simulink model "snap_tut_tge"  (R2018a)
settings: Solver=VariableStepDiscrete  StartTime=0.0  StopTime=50000  RelTol=1e-3
undefined symbols (not defined in the file): bad_frame, Bit, Both, bram, c, cnt_rst, core_rst, d, data, data_in, eof, eof_in, Falling, hex2dec, ip, ip_in, led, led_rx, led_tx, led_up, link_up, Location, Lower, Minimum_Area, notused, out, overrun, reg, Rising, ROACH2, sfp, SNAP, tx_full, tx_over, Unsigned, Upper, valid, valid_in, Width, xc7k160t
libraries: xbsIndex_r4 x1201, casper_library_misc x9, xps_library x5
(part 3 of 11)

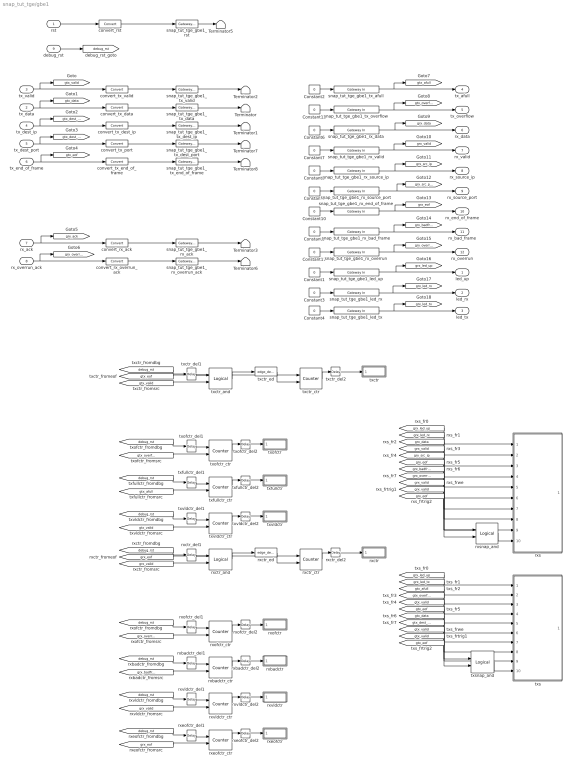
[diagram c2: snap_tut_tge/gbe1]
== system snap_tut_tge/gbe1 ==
  rst : Inport
  tx_data : Inport  Port=2
  tx_valid : Inport  Port=3
  tx_dest_ip : Inport  Port=4
  tx_dest_port : Inport  Port=5
  tx_end_of_frame : Inport  Port=6
  rx_ack : Inport  Port=7
  rx_overrun_ack : Inport  Port=8
  debug_rst : Inport  Port=9
  Constant{1..12} (12 alike) : Constant  Value=0
  Terminator{,1..3,5..8} (8 alike) : Terminator
  convert_rst : xbsIndex_r4/Convert  gui_display_data_type=Fixed-point  arith_type=Boolean  n_bits=64  bin_pt=0  float_type=Single  exp_bits=8  fraction_bits=24  quantization=Truncate  overflow=Wrap  en=off  latency=0  pipeline=off  dbl_ovrd=off  block_type=convert
  convert_rx_ack : xbsIndex_r4/Convert  gui_display_data_type=Fixed-point  arith_type=Boolean  n_bits=64  bin_pt=0  float_type=Single  exp_bits=8  fraction_bits=24  quantization=Truncate  overflow=Wrap  en=off  latency=0  pipeline=off  dbl_ovrd=off  block_type=convert
  convert_rx_overrun_ack : xbsIndex_r4/Convert  gui_display_data_type=Fixed-point  arith_type=Boolean  n_bits=64  bin_pt=0  float_type=Single  exp_bits=8  fraction_bits=24  quantization=Truncate  overflow=Wrap  en=off  latency=0  pipeline=off  dbl_ovrd=off  block_type=convert
  convert_tx_data : xbsIndex_r4/Convert  gui_display_data_type=Fixed-point  arith_type=Unsigned  n_bits=64  bin_pt=0  float_type=Single  exp_bits=8  fraction_bits=24  quantization=Truncate  overflow=Wrap  en=off  latency=0  pipeline=off  dbl_ovrd=off  block_type=convert
  convert_tx_dest_ip : xbsIndex_r4/Convert  gui_display_data_type=Fixed-point  arith_type=Unsigned  n_bits=32  bin_pt=0  float_type=Single  exp_bits=8  fraction_bits=24  quantization=Truncate  overflow=Wrap  en=off  latency=0  pipeline=off  dbl_ovrd=off  block_type=convert
  convert_tx_end_of_frame : xbsIndex_r4/Convert  gui_display_data_type=Fixed-point  arith_type=Boolean  n_bits=1  bin_pt=0  float_type=Single  exp_bits=8  fraction_bits=24  quantization=Truncate  overflow=Wrap  en=off  latency=0  pipeline=off  dbl_ovrd=off  block_type=convert
  convert_tx_port : xbsIndex_r4/Convert  gui_display_data_type=Fixed-point  arith_type=Unsigned  n_bits=16  bin_pt=0  float_type=Single  exp_bits=8  fraction_bits=24  quantization=Truncate  overflow=Wrap  en=off  latency=0  pipeline=off  dbl_ovrd=off  block_type=convert
  convert_tx_valid : xbsIndex_r4/Convert  gui_display_data_type=Fixed-point  arith_type=Boolean  n_bits=1  bin_pt=0  float_type=Single  exp_bits=8  fraction_bits=24  quantization=Truncate  overflow=Wrap  en=off  latency=0  pipeline=off  dbl_ovrd=off  block_type=convert
  rxbadctr : Subsystem  Tag=xps:sw_reg  AncestorBlock=xps_library/Memory/software_register  mask(swreg){io_dir=To Processor, io_delay=1, init_val=0, sample_period=1, names=reg, bitwidths=32, bin_pts=0, arith_types=0, sim_port=off, show_format=on}
      mask prompts: io_dir "I/O direction"; io_delay "I/O delay"; init_val "Initial Value"; sample_period "Sample period"; names "Bitfield names [msb...lsb]"; bitwidths "Bitfield widths"; bin_pts "Bitfield binary pts"; arith_types "Bitfield types, ufix=0, fix=1, bool=2"; sim_port "Provide sim input/output?"; show_format "Print format string?"
      mask help: A 32-bit software-accessible register. Can be divided into bitfields of varying widths and types using the fields in the block mask.
      mask init:
      | swreg_init(gcb)
  rxbadctr_ctr : xbsIndex_r4/Counter  cnt_type=Free Running  cnt_to=Inf  operation=Up  start_count=0  cnt_by_val=1  arith_type=Unsigned  n_bits=32  bin_pt=0  load_pin=off  rst=on  en=on  explicit_period=on  period=1  use_behavioral_HDL=on  implementation=Fabric  dbl_ovrd=off  block_type=counter
  rxbadctr_del1 : xbsIndex_r4/Delay  rst=off  infoeditControl=Selection of Reset will increase slice count due to use of real FFs and instead of SRLs  en=off  latency=2  reg_retiming=on  dbl_ovrd=off  block_type=delay
  rxbadctr_del2 : xbsIndex_r4/Delay  rst=off  infoeditControl=Selection of Reset will increase slice count due to use of real FFs and instead of SRLs  en=off  latency=2  reg_retiming=on  dbl_ovrd=off  block_type=delay
  rxctr : Subsystem  Tag=xps:sw_reg  AncestorBlock=xps_library/Memory/software_register  mask(swreg){io_dir=To Processor, io_delay=1, init_val=0, sample_period=1, names=reg, bitwidths=32, bin_pts=0, arith_types=0, sim_port=off, show_format=on}
      mask prompts: io_dir "I/O direction"; io_delay "I/O delay"; init_val "Initial Value"; sample_period "Sample period"; names "Bitfield names [msb...lsb]"; bitwidths "Bitfield widths"; bin_pts "Bitfield binary pts"; arith_types "Bitfield types, ufix=0, fix=1, bool=2"; sim_port "Provide sim input/output?"; show_format "Print format string?"
      mask help: A 32-bit software-accessible register. Can be divided into bitfields of varying widths and types using the fields in the block mask.
      mask init:
      | swreg_init(gcb)
  rxctr_and : xbsIndex_r4/Logical  logical_function=AND  inputs=2  en=off  latency=1  precision=Full  arith_type=Unsigned  n_bits=16  bin_pt=0  align_bp=on  dbl_ovrd=off  block_type=logical
  rxctr_ctr : xbsIndex_r4/Counter  cnt_type=Free Running  cnt_to=Inf  operation=Up  start_count=0  cnt_by_val=1  arith_type=Unsigned  n_bits=32  bin_pt=0  load_pin=off  rst=on  en=on  explicit_period=on  period=1  use_behavioral_HDL=on  implementation=Fabric  dbl_ovrd=off  block_type=counter
  rxctr_del1 : xbsIndex_r4/Delay  rst=off  infoeditControl=Selection of Reset will increase slice count due to use of real FFs and instead of SRLs  en=off  latency=1  reg_retiming=on  dbl_ovrd=off  block_type=delay
  rxctr_del2 : xbsIndex_r4/Delay  rst=off  infoeditControl=Selection of Reset will increase slice count due to use of real FFs and instead of SRLs  en=off  latency=2  reg_retiming=on  dbl_ovrd=off  block_type=delay
  rxctr_ed : casper_library_misc/edge_detect  edge=Rising  polarity=Active High  x_in=[0 0.08 0.08 0.16 0.16 0.24 0.24 0.32 0.32 0.4]  y_in="[-1 -1  1  1  1  1  1  1  1  1]"  x_out=[0.6 0.68 0.68 0.76 0.76 0.84 0.84 0.92 0.92 1]  y_out="[-1 -1  1  1 -1 -1 -1 -1 -1 -1]"
  rxeofctr : Subsystem  Tag=xps:sw_reg  AncestorBlock=xps_library/Memory/software_register  mask(swreg){io_dir=To Processor, io_delay=1, init_val=0, sample_period=1, names=reg, bitwidths=32, bin_pts=0, arith_types=0, sim_port=off, show_format=on}
      mask prompts: io_dir "I/O direction"; io_delay "I/O delay"; init_val "Initial Value"; sample_period "Sample period"; names "Bitfield names [msb...lsb]"; bitwidths "Bitfield widths"; bin_pts "Bitfield binary pts"; arith_types "Bitfield types, ufix=0, fix=1, bool=2"; sim_port "Provide sim input/output?"; show_format "Print format string?"
      mask help: A 32-bit software-accessible register. Can be divided into bitfields of varying widths and types using the fields in the block mask.
      mask init:
      | swreg_init(gcb)
  rxeofctr_ctr : xbsIndex_r4/Counter  cnt_type=Free Running  cnt_to=Inf  operation=Up  start_count=0  cnt_by_val=1  arith_type=Unsigned  n_bits=32  bin_pt=0  load_pin=off  rst=on  en=on  explicit_period=on  period=1  use_behavioral_HDL=on  implementation=Fabric  dbl_ovrd=off  block_type=counter
  rxeofctr_del1 : xbsIndex_r4/Delay  rst=off  infoeditControl=Selection of Reset will increase slice count due to use of real FFs and instead of SRLs  en=off  latency=2  reg_retiming=on  dbl_ovrd=off  block_type=delay
  rxeofctr_del2 : xbsIndex_r4/Delay  rst=off  infoeditControl=Selection of Reset will increase slice count due to use of real FFs and instead of SRLs  en=off  latency=2  reg_retiming=on  dbl_ovrd=off  block_type=delay
  rxofctr : Subsystem  Tag=xps:sw_reg  AncestorBlock=xps_library/Memory/software_register  mask(swreg){io_dir=To Processor, io_delay=1, init_val=0, sample_period=1, names=reg, bitwidths=32, bin_pts=0, arith_types=0, sim_port=off, show_format=on}
      mask prompts: io_dir "I/O direction"; io_delay "I/O delay"; init_val "Initial Value"; sample_period "Sample period"; names "Bitfield names [msb...lsb]"; bitwidths "Bitfield widths"; bin_pts "Bitfield binary pts"; arith_types "Bitfield types, ufix=0, fix=1, bool=2"; sim_port "Provide sim input/output?"; show_format "Print format string?"
      mask help: A 32-bit software-accessible register. Can be divided into bitfields of varying widths and types using the fields in the block mask.
      mask init:
      | swreg_init(gcb)
  rxofctr_ctr : xbsIndex_r4/Counter  cnt_type=Free Running  cnt_to=Inf  operation=Up  start_count=0  cnt_by_val=1  arith_type=Unsigned  n_bits=32  bin_pt=0  load_pin=off  rst=on  en=on  explicit_period=on  period=1  use_behavioral_HDL=on  implementation=Fabric  dbl_ovrd=off  block_type=counter
  rxofctr_del1 : xbsIndex_r4/Delay  rst=off  infoeditControl=Selection of Reset will increase slice count due to use of real FFs and instead of SRLs  en=off  latency=2  reg_retiming=on  dbl_ovrd=off  block_type=delay
  rxofctr_del2 : xbsIndex_r4/Delay  rst=off  infoeditControl=Selection of Reset will increase slice count due to use of real FFs and instead of SRLs  en=off  latency=2  reg_retiming=on  dbl_ovrd=off  block_type=delay
  rxs : Subsystem  Tag=casper:bitsnap  AncestorBlock=casper_library_scopes/bitfield_snapshot  mask(bitsnap){io_names=[led_up led_rx data_in valid_in ip_in eof_in bad_frame overrun], io_widths=[1 1 64 1 32 1 1 1], io_bps=[0 0 0 0 0 0 0 0], io_types=[2 2 0 2 0 2 2 2], show_format=on, snap_storage=bram, snap_dram_dimm=2, snap_dram_clock=250, snap_nsamples=13, snap_data_width=128, snap_offset=off, snap_circap=off, snap_value=off, snap_ext_arm=off, snap_ext_circ=off, snap_provide_outputs=on, snap_use_dsp48=on, snap_delay=5, extra_names=[notused], extra_widths=[32], extra_bps=[0], extra_types=[0]}
      mask prompts: io_names "Names [msb...lsb]"; io_widths "Bitwidths [msb...lsb]"; io_bps "Binary pts [msb...lsb]"; io_types "Data types [msb...lsb], ufix=0, fix=1, bool=2"; show_format "Print format string?"; snap_storage "Storage medium"; snap_dram_dimm "DRAM dimm"; snap_dram_clock "DRAM clock rate"; snap_nsamples "Number of Samples (2^?)"; snap_data_width "Data width"; snap_offset "Start delay support"; snap_circap "Circular capture support"; snap_value "Extra value capture support"; snap_ext_arm "External arm support"; snap_ext_circ "External circular capture support"; snap_provide_outputs "Provide outputs"; snap_use_dsp48 "Use DSP48s to implement counters"; snap_delay "Pre-snapshot delay"; extra_names "Names [msb...lsb]"; extra_widths "Widths [msb...lsb]"; extra_bps "Binary pts [msb...lsb]"; extra_types "Data types [msb...lsb], ufix=0, fix=1, bool=2"
      mask help: A wrapped snapshot block. Allows specification of inputs to a snapblock word so the toolflow can automatically set up the scope. See documentation for snapshot for explanation of parameters.
      mask init:
      | bitsnap_init(gcb);
  rxsnap_and : xbsIndex_r4/Logical  logical_function=AND  inputs=2  en=off  latency=1  precision=Full  arith_type=Unsigned  n_bits=16  bin_pt=0  align_bp=on  dbl_ovrd=off  block_type=logical
  rxvldctr : Subsystem  Tag=xps:sw_reg  AncestorBlock=xps_library/Memory/software_register  mask(swreg){io_dir=To Processor, io_delay=1, init_val=0, sample_period=1, names=reg, bitwidths=32, bin_pts=0, arith_types=0, sim_port=off, show_format=on}
      mask prompts: io_dir "I/O direction"; io_delay "I/O delay"; init_val "Initial Value"; sample_period "Sample period"; names "Bitfield names [msb...lsb]"; bitwidths "Bitfield widths"; bin_pts "Bitfield binary pts"; arith_types "Bitfield types, ufix=0, fix=1, bool=2"; sim_port "Provide sim input/output?"; show_format "Print format string?"
      mask help: A 32-bit software-accessible register. Can be divided into bitfields of varying widths and types using the fields in the block mask.
      mask init:
      | swreg_init(gcb)
  rxvldctr_ctr : xbsIndex_r4/Counter  cnt_type=Free Running  cnt_to=Inf  operation=Up  start_count=0  cnt_by_val=1  arith_type=Unsigned  n_bits=32  bin_pt=0  load_pin=off  rst=on  en=on  explicit_period=on  period=1  use_behavioral_HDL=on  implementation=Fabric  dbl_ovrd=off  block_type=counter
  rxvldctr_del1 : xbsIndex_r4/Delay  rst=off  infoeditControl=Selection of Reset will increase slice count due to use of real FFs and instead of SRLs  en=off  latency=2  reg_retiming=on  dbl_ovrd=off  block_type=delay
  rxvldctr_del2 : xbsIndex_r4/Delay  rst=off  infoeditControl=Selection of Reset will increase slice count due to use of real FFs and instead of SRLs  en=off  latency=2  reg_retiming=on  dbl_ovrd=off  block_type=delay
  snap_tut_tge_gbe1_led_rx : xbsIndex_r4/Gateway In  gui_display_data_type=Fixed-point  arith_type=Boolean  n_bits=1  bin_pt=0  preci_type=Single  exp_width=8  frac_width=24  rows=1  columns=1  quantization=Truncate  overflow=Wrap  period=1  UseAsADC=off  ADCChannel='1'  interface=None  automatic_assignment=on  address_offset=hex2dec('00')  intf_name=''  intf_description=''  default_value=0  timing_constraint=None  locs_specified=off  LOCs={}  io_standard={}  inherit_from_input=off  hdl_port=on  dbl_ovrd=off  block_type=gatewayin
  snap_tut_tge_gbe1_led_tx : xbsIndex_r4/Gateway In  gui_display_data_type=Fixed-point  arith_type=Boolean  n_bits=1  bin_pt=0  preci_type=Single  exp_width=8  frac_width=24  rows=1  columns=1  quantization=Truncate  overflow=Wrap  period=1  UseAsADC=off  ADCChannel='1'  interface=None  automatic_assignment=on  address_offset=hex2dec('00')  intf_name=''  intf_description=''  default_value=0  timing_constraint=None  locs_specified=off  LOCs={}  io_standard={}  inherit_from_input=off  hdl_port=on  dbl_ovrd=off  block_type=gatewayin
  snap_tut_tge_gbe1_led_up : xbsIndex_r4/Gateway In  gui_display_data_type=Fixed-point  arith_type=Boolean  n_bits=1  bin_pt=0  preci_type=Single  exp_width=8  frac_width=24  rows=1  columns=1  quantization=Truncate  overflow=Wrap  period=1  UseAsADC=off  ADCChannel='1'  interface=None  automatic_assignment=on  address_offset=hex2dec('00')  intf_name=''  intf_description=''  default_value=0  timing_constraint=None  locs_specified=off  LOCs={}  io_standard={}  inherit_from_input=off  hdl_port=on  dbl_ovrd=off  block_type=gatewayin
  snap_tut_tge_gbe1_rst : xbsIndex_r4/Gateway Out  inherit_from_input=off  hdl_port=on  rows=1  columns=1  UseAsDAC=off  DACChannel='1'  interface=None  automatic_assignment=on  address_offset=hex2dec('00')  intf_name=''  intf_description=''  timing_constraint=None  locs_specified=off  LOCs={}  io_standard={}  block_type=gatewayout
  snap_tut_tge_gbe1_rx_ack : xbsIndex_r4/Gateway Out  inherit_from_input=off  hdl_port=on  rows=1  columns=1  UseAsDAC=off  DACChannel='1'  interface=None  automatic_assignment=on  address_offset=hex2dec('00')  intf_name=''  intf_description=''  timing_constraint=None  locs_specified=off  LOCs={}  io_standard={}  block_type=gatewayout
  snap_tut_tge_gbe1_rx_bad_frame : xbsIndex_r4/Gateway In  gui_display_data_type=Fixed-point  arith_type=Boolean  n_bits=1  bin_pt=0  preci_type=Single  exp_width=8  frac_width=24  rows=1  columns=1  quantization=Truncate  overflow=Wrap  period=1  UseAsADC=off  ADCChannel='1'  interface=None  automatic_assignment=on  address_offset=hex2dec('00')  intf_name=''  intf_description=''  default_value=0  timing_constraint=None  locs_specified=off  LOCs={}  io_standard={}  inherit_from_input=off  hdl_port=on  dbl_ovrd=off  block_type=gatewayin
  snap_tut_tge_gbe1_rx_data : xbsIndex_r4/Gateway In  gui_display_data_type=Fixed-point  arith_type=Unsigned  n_bits=64  bin_pt=0  preci_type=Single  exp_width=8  frac_width=24  rows=1  columns=1  quantization=Truncate  overflow=Wrap  period=1  UseAsADC=off  ADCChannel='1'  interface=None  automatic_assignment=on  address_offset=hex2dec('00')  intf_name=''  intf_description=''  default_value=0  timing_constraint=None  locs_specified=off  LOCs={}  io_standard={}  inherit_from_input=off  hdl_port=on  dbl_ovrd=off  block_type=gatewayin
  snap_tut_tge_gbe1_rx_end_of_frame : xbsIndex_r4/Gateway In  gui_display_data_type=Fixed-point  arith_type=Boolean  n_bits=1  bin_pt=0  preci_type=Single  exp_width=8  frac_width=24  rows=1  columns=1  quantization=Truncate  overflow=Wrap  period=1  UseAsADC=off  ADCChannel='1'  interface=None  automatic_assignment=on  address_offset=hex2dec('00')  intf_name=''  intf_description=''  default_value=0  timing_constraint=None  locs_specified=off  LOCs={}  io_standard={}  inherit_from_input=off  hdl_port=on  dbl_ovrd=off  block_type=gatewayin
  snap_tut_tge_gbe1_rx_overrun : xbsIndex_r4/Gateway In  gui_display_data_type=Fixed-point  arith_type=Boolean  n_bits=1  bin_pt=0  preci_type=Single  exp_width=8  frac_width=24  rows=1  columns=1  quantization=Truncate  overflow=Wrap  period=1  UseAsADC=off  ADCChannel='1'  interface=None  automatic_assignment=on  address_offset=hex2dec('00')  intf_name=''  intf_description=''  default_value=0  timing_constraint=None  locs_specified=off  LOCs={}  io_standard={}  inherit_from_input=off  hdl_port=on  dbl_ovrd=off  block_type=gatewayin
  snap_tut_tge_gbe1_rx_overrun_ack : xbsIndex_r4/Gateway Out  inherit_from_input=off  hdl_port=on  rows=1  columns=1  UseAsDAC=off  DACChannel='1'  interface=None  automatic_assignment=on  address_offset=hex2dec('00')  intf_name=''  intf_description=''  timing_constraint=None  locs_specified=off  LOCs={}  io_standard={}  block_type=gatewayout
  snap_tut_tge_gbe1_rx_source_ip : xbsIndex_r4/Gateway In  gui_display_data_type=Fixed-point  arith_type=Unsigned  n_bits=32  bin_pt=0  preci_type=Single  exp_width=8  frac_width=24  rows=1  columns=1  quantization=Truncate  overflow=Wrap  period=1  UseAsADC=off  ADCChannel='1'  interface=None  automatic_assignment=on  address_offset=hex2dec('00')  intf_name=''  intf_description=''  default_value=0  timing_constraint=None  locs_specified=off  LOCs={}  io_standard={}  inherit_from_input=off  hdl_port=on  dbl_ovrd=off  block_type=gatewayin
  snap_tut_tge_gbe1_rx_source_port : xbsIndex_r4/Gateway In  gui_display_data_type=Fixed-point  arith_type=Unsigned  n_bits=16  bin_pt=0  preci_type=Single  exp_width=8  frac_width=24  rows=1  columns=1  quantization=Truncate  overflow=Wrap  period=1  UseAsADC=off  ADCChannel='1'  interface=None  automatic_assignment=on  address_offset=hex2dec('00')  intf_name=''  intf_description=''  default_value=0  timing_constraint=None  locs_specified=off  LOCs={}  io_standard={}  inherit_from_input=off  hdl_port=on  dbl_ovrd=off  block_type=gatewayin
  snap_tut_tge_gbe1_rx_valid : xbsIndex_r4/Gateway In  gui_display_data_type=Fixed-point  arith_type=Boolean  n_bits=1  bin_pt=0  preci_type=Single  exp_width=8  frac_width=24  rows=1  columns=1  quantization=Truncate  overflow=Wrap  period=1  UseAsADC=off  ADCChannel='1'  interface=None  automatic_assignment=on  address_offset=hex2dec('00')  intf_name=''  intf_description=''  default_value=0  timing_constraint=None  locs_specified=off  LOCs={}  io_standard={}  inherit_from_input=off  hdl_port=on  dbl_ovrd=off  block_type=gatewayin
  snap_tut_tge_gbe1_tx_afull : xbsIndex_r4/Gateway In  gui_display_data_type=Fixed-point  arith_type=Boolean  n_bits=1  bin_pt=0  preci_type=Single  exp_width=8  frac_width=24  rows=1  columns=1  quantization=Truncate  overflow=Wrap  period=1  UseAsADC=off  ADCChannel='1'  interface=None  automatic_assignment=on  address_offset=hex2dec('00')  intf_name=''  intf_description=''  default_value=0  timing_constraint=None  locs_specified=off  LOCs={}  io_standard={}  inherit_from_input=off  hdl_port=on  dbl_ovrd=off  block_type=gatewayin
  snap_tut_tge_gbe1_tx_data : xbsIndex_r4/Gateway Out  inherit_from_input=off  hdl_port=on  rows=1  columns=1  UseAsDAC=off  DACChannel='1'  interface=None  automatic_assignment=on  address_offset=hex2dec('00')  intf_name=''  intf_description=''  timing_constraint=None  locs_specified=off  LOCs={}  io_standard={}  block_type=gatewayout
  snap_tut_tge_gbe1_tx_dest_ip : xbsIndex_r4/Gateway Out  inherit_from_input=off  hdl_port=on  rows=1  columns=1  UseAsDAC=off  DACChannel='1'  interface=None  automatic_assignment=on  address_offset=hex2dec('00')  intf_name=''  intf_description=''  timing_constraint=None  locs_specified=off  LOCs={}  io_standard={}  block_type=gatewayout
  snap_tut_tge_gbe1_tx_dest_port : xbsIndex_r4/Gateway Out  inherit_from_input=off  hdl_port=on  rows=1  columns=1  UseAsDAC=off  DACChannel='1'  interface=None  automatic_assignment=on  address_offset=hex2dec('00')  intf_name=''  intf_description=''  timing_constraint=None  locs_specified=off  LOCs={}  io_standard={}  block_type=gatewayout
  snap_tut_tge_gbe1_tx_end_of_frame : xbsIndex_r4/Gateway Out  inherit_from_input=off  hdl_port=on  rows=1  columns=1  UseAsDAC=off  DACChannel='1'  interface=None  automatic_assignment=on  address_offset=hex2dec('00')  intf_name=''  intf_description=''  timing_constraint=None  locs_specified=off  LOCs={}  io_standard={}  block_type=gatewayout
  snap_tut_tge_gbe1_tx_overflow : xbsIndex_r4/Gateway In  gui_display_data_type=Fixed-point  arith_type=Boolean  n_bits=1  bin_pt=0  preci_type=Single  exp_width=8  frac_width=24  rows=1  columns=1  quantization=Truncate  overflow=Wrap  period=1  UseAsADC=off  ADCChannel='1'  interface=None  automatic_assignment=on  address_offset=hex2dec('00')  intf_name=''  intf_description=''  default_value=0  timing_constraint=None  locs_specified=off  LOCs={}  io_standard={}  inherit_from_input=off  hdl_port=on  dbl_ovrd=off  block_type=gatewayin
  snap_tut_tge_gbe1_tx_valid : xbsIndex_r4/Gateway Out  inherit_from_input=off  hdl_port=on  rows=1  columns=1  UseAsDAC=off  DACChannel='1'  interface=None  automatic_assignment=on  address_offset=hex2dec('00')  intf_name=''  intf_description=''  timing_constraint=None  locs_specified=off  LOCs={}  io_standard={}  block_type=gatewayout
  txctr : Subsystem  Tag=xps:sw_reg  AncestorBlock=xps_library/Memory/software_register  mask(swreg){io_dir=To Processor, io_delay=1, init_val=0, sample_period=1, names=reg, bitwidths=32, bin_pts=0, arith_types=0, sim_port=off, show_format=on}
      mask prompts: io_dir "I/O direction"; io_delay "I/O delay"; init_val "Initial Value"; sample_period "Sample period"; names "Bitfield names [msb...lsb]"; bitwidths "Bitfield widths"; bin_pts "Bitfield binary pts"; arith_types "Bitfield types, ufix=0, fix=1, bool=2"; sim_port "Provide sim input/output?"; show_format "Print format string?"
      mask help: A 32-bit software-accessible register. Can be divided into bitfields of varying widths and types using the fields in the block mask.
      mask init:
      | swreg_init(gcb)
  txctr_and : xbsIndex_r4/Logical  logical_function=AND  inputs=2  en=off  latency=1  precision=Full  arith_type=Unsigned  n_bits=16  bin_pt=0  align_bp=on  dbl_ovrd=off  block_type=logical
  txctr_ctr : xbsIndex_r4/Counter  cnt_type=Free Running  cnt_to=Inf  operation=Up  start_count=0  cnt_by_val=1  arith_type=Unsigned  n_bits=32  bin_pt=0  load_pin=off  rst=on  en=on  explicit_period=on  period=1  use_behavioral_HDL=on  implementation=Fabric  dbl_ovrd=off  block_type=counter
  txctr_del1 : xbsIndex_r4/Delay  rst=off  infoeditControl=Selection of Reset will increase slice count due to use of real FFs and instead of SRLs  en=off  latency=1  reg_retiming=on  dbl_ovrd=off  block_type=delay
  txctr_del2 : xbsIndex_r4/Delay  rst=off  infoeditControl=Selection of Reset will increase slice count due to use of real FFs and instead of SRLs  en=off  latency=2  reg_retiming=on  dbl_ovrd=off  block_type=delay
  txctr_ed : casper_library_misc/edge_detect  edge=Rising  polarity=Active High  x_in=[0 0.08 0.08 0.16 0.16 0.24 0.24 0.32 0.32 0.4]  y_in="[-1 -1  1  1  1  1  1  1  1  1]"  x_out=[0.6 0.68 0.68 0.76 0.76 0.84 0.84 0.92 0.92 1]  y_out="[-1 -1  1  1 -1 -1 -1 -1 -1 -1]"
  txfullctr : Subsystem  Tag=xps:sw_reg  AncestorBlock=xps_library/Memory/software_register  mask(swreg){io_dir=To Processor, io_delay=1, init_val=0, sample_period=1, names=reg, bitwidths=32, bin_pts=0, arith_types=0, sim_port=off, show_format=on}
      mask prompts: io_dir "I/O direction"; io_delay "I/O delay"; init_val "Initial Value"; sample_period "Sample period"; names "Bitfield names [msb...lsb]"; bitwidths "Bitfield widths"; bin_pts "Bitfield binary pts"; arith_types "Bitfield types, ufix=0, fix=1, bool=2"; sim_port "Provide sim input/output?"; show_format "Print format string?"
      mask help: A 32-bit software-accessible register. Can be divided into bitfields of varying widths and types using the fields in the block mask.
      mask init:
      | swreg_init(gcb)
  txfullctr_ctr : xbsIndex_r4/Counter  cnt_type=Free Running  cnt_to=Inf  operation=Up  start_count=0  cnt_by_val=1  arith_type=Unsigned  n_bits=32  bin_pt=0  load_pin=off  rst=on  en=on  explicit_period=on  period=1  use_behavioral_HDL=on  implementation=Fabric  dbl_ovrd=off  block_type=counter
  txfullctr_del1 : xbsIndex_r4/Delay  rst=off  infoeditControl=Selection of Reset will increase slice count due to use of real FFs and instead of SRLs  en=off  latency=2  reg_retiming=on  dbl_ovrd=off  block_type=delay
  txfullctr_del2 : xbsIndex_r4/Delay  rst=off  infoeditControl=Selection of Reset will increase slice count due to use of real FFs and instead of SRLs  en=off  latency=2  reg_retiming=on  dbl_ovrd=off  block_type=delay
  txofctr : Subsystem  Tag=xps:sw_reg  AncestorBlock=xps_library/Memory/software_register  mask(swreg){io_dir=To Processor, io_delay=1, init_val=0, sample_period=1, names=reg, bitwidths=32, bin_pts=0, arith_types=0, sim_port=off, show_format=on}
      mask prompts: io_dir "I/O direction"; io_delay "I/O delay"; init_val "Initial Value"; sample_period "Sample period"; names "Bitfield names [msb...lsb]"; bitwidths "Bitfield widths"; bin_pts "Bitfield binary pts"; arith_types "Bitfield types, ufix=0, fix=1, bool=2"; sim_port "Provide sim input/output?"; show_format "Print format string?"
      mask help: A 32-bit software-accessible register. Can be divided into bitfields of varying widths and types using the fields in the block mask.
      mask init:
      | swreg_init(gcb)
  txofctr_ctr : xbsIndex_r4/Counter  cnt_type=Free Running  cnt_to=Inf  operation=Up  start_count=0  cnt_by_val=1  arith_type=Unsigned  n_bits=32  bin_pt=0  load_pin=off  rst=on  en=on  explicit_period=on  period=1  use_behavioral_HDL=on  implementation=Fabric  dbl_ovrd=off  block_type=counter
  txofctr_del1 : xbsIndex_r4/Delay  rst=off  infoeditControl=Selection of Reset will increase slice count due to use of real FFs and instead of SRLs  en=off  latency=2  reg_retiming=on  dbl_ovrd=off  block_type=delay
  txofctr_del2 : xbsIndex_r4/Delay  rst=off  infoeditControl=Selection of Reset will increase slice count due to use of real FFs and instead of SRLs  en=off  latency=2  reg_retiming=on  dbl_ovrd=off  block_type=delay
  txs : Subsystem  Tag=casper:bitsnap  AncestorBlock=casper_library_scopes/bitfield_snapshot  mask(bitsnap){io_names=[link_up led_tx tx_full tx_over valid eof data ip], io_widths=[1 1 1 1 1 1 64 32], io_bps=[0 0 0 0 0 0 0 0], io_types=[2 2 2 2 2 2 0 0], show_format=on, snap_storage=bram, snap_dram_dimm=2, snap_dram_clock=250, snap_nsamples=13, snap_data_width=128, snap_offset=off, snap_circap=off, snap_value=off, snap_ext_arm=off, snap_ext_circ=off, snap_provide_outputs=on, snap_use_dsp48=on, snap_delay=5, extra_names=[notused], extra_widths=[32], extra_bps=[0], extra_types=[0]}
      mask prompts: io_names "Names [msb...lsb]"; io_widths "Bitwidths [msb...lsb]"; io_bps "Binary pts [msb...lsb]"; io_types "Data types [msb...lsb], ufix=0, fix=1, bool=2"; show_format "Print format string?"; snap_storage "Storage medium"; snap_dram_dimm "DRAM dimm"; snap_dram_clock "DRAM clock rate"; snap_nsamples "Number of Samples (2^?)"; snap_data_width "Data width"; snap_offset "Start delay support"; snap_circap "Circular capture support"; snap_value "Extra value capture support"; snap_ext_arm "External arm support"; snap_ext_circ "External circular capture support"; snap_provide_outputs "Provide outputs"; snap_use_dsp48 "Use DSP48s to implement counters"; snap_delay "Pre-snapshot delay"; extra_names "Names [msb...lsb]"; extra_widths "Widths [msb...lsb]"; extra_bps "Binary pts [msb...lsb]"; extra_types "Data types [msb...lsb], ufix=0, fix=1, bool=2"
      mask help: A wrapped snapshot block. Allows specification of inputs to a snapblock word so the toolflow can automatically set up the scope. See documentation for snapshot for explanation of parameters.
      mask init:
      | bitsnap_init(gcb);
  txsnap_and : xbsIndex_r4/Logical  logical_function=AND  inputs=2  en=off  latency=1  precision=Full  arith_type=Unsigned  n_bits=16  bin_pt=0  align_bp=on  dbl_ovrd=off  block_type=logical
  txvldctr : Subsystem  Tag=xps:sw_reg  AncestorBlock=xps_library/Memory/software_register  mask(swreg){io_dir=To Processor, io_delay=1, init_val=0, sample_period=1, names=reg, bitwidths=32, bin_pts=0, arith_types=0, sim_port=off, show_format=on}
      mask prompts: io_dir "I/O direction"; io_delay "I/O delay"; init_val "Initial Value"; sample_period "Sample period"; names "Bitfield names [msb...lsb]"; bitwidths "Bitfield widths"; bin_pts "Bitfield binary pts"; arith_types "Bitfield types, ufix=0, fix=1, bool=2"; sim_port "Provide sim input/output?"; show_format "Print format string?"
      mask help: A 32-bit software-accessible register. Can be divided into bitfields of varying widths and types using the fields in the block mask.
      mask init:
      | swreg_init(gcb)
  txvldctr_ctr : xbsIndex_r4/Counter  cnt_type=Free Running  cnt_to=Inf  operation=Up  start_count=0  cnt_by_val=1  arith_type=Unsigned  n_bits=32  bin_pt=0  load_pin=off  rst=on  en=on  explicit_period=on  period=1  use_behavioral_HDL=on  implementation=Fabric  dbl_ovrd=off  block_type=counter
  txvldctr_del1 : xbsIndex_r4/Delay  rst=off  infoeditControl=Selection of Reset will increase slice count due to use of real FFs and instead of SRLs  en=off  latency=2  reg_retiming=on  dbl_ovrd=off  block_type=delay
  txvldctr_del2 : xbsIndex_r4/Delay  rst=off  infoeditControl=Selection of Reset will increase slice count due to use of real FFs and instead of SRLs  en=off  latency=2  reg_retiming=on  dbl_ovrd=off  block_type=delay
  led_up : Outport
  led_rx : Outport  Port=2
  led_tx : Outport  Port=3
  tx_afull : Outport  Port=4
  tx_overflow : Outport  Port=5
  rx_data : Outport  Port=6
  rx_valid : Outport  Port=7
  rx_source_ip : Outport  Port=8
  rx_source_port : Outport  Port=9
  rx_end_of_frame : Outport  Port=10
  rx_bad_frame : Outport  Port=11
  rx_overrun : Outport  Port=12
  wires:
  snap_tut_tge_gbe1_led_tx/1 -> led_tx/1, [grx_led_tx]
  Constant4/1 -> snap_tut_tge_gbe1_led_tx/1
  snap_tut_tge_gbe1_led_rx/1 -> led_rx/1, [grx_led_rx]
  Constant3/1 -> snap_tut_tge_gbe1_led_rx/1
  snap_tut_tge_gbe1_led_up/1 -> led_up/1, [grx_led_up]
  Constant1/1 -> snap_tut_tge_gbe1_led_up/1
  snap_tut_tge_gbe1_rx_end_of_frame/1 -> rx_end_of_frame/1, [grx_eof]
  Constant10/1 -> snap_tut_tge_gbe1_rx_end_of_frame/1
  snap_tut_tge_gbe1_rx_source_port/1 -> rx_source_port/1, [grx_src_port]
  Constant9/1 -> snap_tut_tge_gbe1_rx_source_port/1
  Constant8/1 -> snap_tut_tge_gbe1_rx_source_ip/1
  snap_tut_tge_gbe1_rx_source_ip/1 -> rx_source_ip/1, [grx_src_ip]
  snap_tut_tge_gbe1_tx_end_of_frame/1 -> Terminator8/1
  convert_tx_end_of_frame/1 -> snap_tut_tge_gbe1_tx_end_of_frame/1
  tx_end_of_frame/1 -> convert_tx_end_of_frame/1, [gtx_eof]
  snap_tut_tge_gbe1_tx_dest_port/1 -> Terminator7/1
  convert_tx_port/1 -> snap_tut_tge_gbe1_tx_dest_port/1
  tx_dest_port/1 -> convert_tx_port/1, [gtx_dest_port]
  snap_tut_tge_gbe1_rst/1 -> Terminator5/1
  convert_rst/1 -> snap_tut_tge_gbe1_rst/1
  rst/1 -> convert_rst/1
  snap_tut_tge_gbe1_rx_valid/1 -> rx_valid/1, [grx_valid]
  Constant7/1 -> snap_tut_tge_gbe1_rx_valid/1
  snap_tut_tge_gbe1_rx_ack/1 -> Terminator3/1
  Constant6/1 -> snap_tut_tge_gbe1_rx_data/1
  Constant2/1 -> snap_tut_tge_gbe1_tx_afull/1
  snap_tut_tge_gbe1_tx_valid/1 -> Terminator2/1
  snap_tut_tge_gbe1_tx_dest_ip/1 -> Terminator1/1
  snap_tut_tge_gbe1_tx_data/1 -> Terminator/1
  snap_tut_tge_gbe1_tx_afull/1 -> tx_afull/1, [gtx_afull]
  convert_tx_valid/1 -> snap_tut_tge_gbe1_tx_valid/1
  tx_valid/1 -> convert_tx_valid/1, [gtx_valid]
  convert_tx_dest_ip/1 -> snap_tut_tge_gbe1_tx_dest_ip/1
  tx_dest_ip/1 -> convert_tx_dest_ip/1, [gtx_dest_ip]
  convert_tx_data/1 -> snap_tut_tge_gbe1_tx_data/1
  tx_data/1 -> convert_tx_data/1, [gtx_data]
  snap_tut_tge_gbe1_rx_data/1 -> rx_data/1, [grx_data]
  convert_rx_ack/1 -> snap_tut_tge_gbe1_rx_ack/1
  rx_ack/1 -> convert_rx_ack/1, [grx_ack]
  snap_tut_tge_gbe1_rx_bad_frame/1 -> rx_bad_frame/1, [grx_badframe]
  Constant5/1 -> snap_tut_tge_gbe1_rx_bad_frame/1
  snap_tut_tge_gbe1_rx_overrun/1 -> rx_overrun/1, [grx_overrun]
  Constant11/1 -> snap_tut_tge_gbe1_rx_overrun/1
  snap_tut_tge_gbe1_rx_overrun_ack/1 -> Terminator6/1
  convert_rx_overrun_ack/1 -> snap_tut_tge_gbe1_rx_overrun_ack/1
  rx_overrun_ack/1 -> convert_rx_overrun_ack/1, [grx_overrun_ack]
  Constant12/1 -> snap_tut_tge_gbe1_tx_overflow/1
  snap_tut_tge_gbe1_tx_overflow/1 -> tx_overflow/1, [gtx_overflow]
  debug_rst/1 -> [debug_rst]
  [gtx_eof] -> txctr_and/1
  [gtx_valid] -> txctr_and/2
  txctr_and/1 -> txctr_ed/1
  [debug_rst] -> txctr_del1/1
  txctr_del1/1 -> txctr_ctr/1
  txctr_ed/1 -> txctr_ctr/2
  txctr_ctr/1 -> txctr_del2/1
  txctr_del2/1 -> txctr/1(out_reg)
  [debug_rst] -> txofctr_del1/1
  txofctr_del1/1 -> txofctr_ctr/1
  [gtx_overflow] -> txofctr_ctr/2
  txofctr_ctr/1 -> txofctr_del2/1
  txofctr_del2/1 -> txofctr/1(out_reg)
  [debug_rst] -> txfullctr_del1/1
  txfullctr_del1/1 -> txfullctr_ctr/1
  [gtx_afull] -> txfullctr_ctr/2
  txfullctr_ctr/1 -> txfullctr_del2/1
  txfullctr_del2/1 -> txfullctr/1(out_reg)
  [debug_rst] -> txvldctr_del1/1
  txvldctr_del1/1 -> txvldctr_ctr/1
  [gtx_valid] -> txvldctr_ctr/2
  txvldctr_ctr/1 -> txvldctr_del2/1
  txvldctr_del2/1 -> txvldctr/1(out_reg)
  [grx_eof] -> rxctr_and/1
  [grx_valid] -> rxctr_and/2
  rxctr_and/1 -> rxctr_ed/1
  [debug_rst] -> rxctr_del1/1
  rxctr_del1/1 -> rxctr_ctr/1
  rxctr_ed/1 -> rxctr_ctr/2
  rxctr_ctr/1 -> rxctr_del2/1
  rxctr_del2/1 -> rxctr/1(out_reg)
  [debug_rst] -> rxofctr_del1/1
  rxofctr_del1/1 -> rxofctr_ctr/1
  [grx_overrun] -> rxofctr_ctr/2
  rxofctr_ctr/1 -> rxofctr_del2/1
  rxofctr_del2/1 -> rxofctr/1(out_reg)
  [debug_rst] -> rxbadctr_del1/1
  rxbadctr_del1/1 -> rxbadctr_ctr/1
  [grx_badframe] -> rxbadctr_ctr/2
  rxbadctr_ctr/1 -> rxbadctr_del2/1
  rxbadctr_del2/1 -> rxbadctr/1(out_reg)
  [debug_rst] -> rxvldctr_del1/1
  rxvldctr_del1/1 -> rxvldctr_ctr/1
  [grx_valid] -> rxvldctr_ctr/2
  rxvldctr_ctr/1 -> rxvldctr_del2/1
  rxvldctr_del2/1 -> rxvldctr/1(out_reg)
  [debug_rst] -> rxeofctr_del1/1
  rxeofctr_del1/1 -> rxeofctr_ctr/1
  [grx_eof] -> rxeofctr_ctr/2
  rxeofctr_ctr/1 -> rxeofctr_del2/1
  rxeofctr_del2/1 -> rxeofctr/1(out_reg)
  [grx_led_rx] -> rxs/2(in_led_rx)
  [grx_eof] -> rxs/6(in_eof_in)
  [grx_valid] -> rxs/9(we)
  [gtx_eof] -> txs/6(in_eof)
  [gtx_valid] -> txs/9(we)
  [grx_led_up] -> rxs/1(in_led_up)
  [grx_data] -> rxs/3(in_data_in)
  [grx_valid] -> rxs/4(in_valid_in)
  [grx_src_ip] -> rxs/5(in_ip_in)
  [grx_badframe] -> rxs/7(in_bad_frame)
  [grx_overrun] -> rxs/8(in_overrun)
  [grx_valid] -> rxsnap_and/1
  [grx_eof] -> rxsnap_and/2
  rxsnap_and/1 -> rxs/10(trig)
  [grx_led_up] -> txs/1(in_link_up)
  [grx_led_tx] -> txs/2(in_led_tx)
  [gtx_afull] -> txs/3(in_tx_full)
  [gtx_overflow] -> txs/4(in_tx_over)
  [gtx_valid] -> txs/5(in_valid)
  [gtx_data] -> txs/7(in_data)
  [gtx_dest_ip] -> txs/8(in_ip)
  [gtx_valid] -> txsnap_and/1
  [gtx_eof] -> txsnap_and/2
  txsnap_and/1 -> txs/10(trig)

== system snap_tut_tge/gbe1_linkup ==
  out_reg : Inport
  assert_reg : xbsIndex_r4/Assert  assert_type=on  type_source=Explicitly  gui_display_data_type=Boolean  arith_type=Boolean  n_bits=1  bin_pt=0  preci_type=Single  exp_width=8  frac_width=24  assert_rate=off  rate_source=Explicitly  period=1  output_port=on  block_type=assert
  cast_gw : xbsIndex_r4/Convert  gui_display_data_type=Fixed-point  arith_type=Unsigned  n_bits=32  bin_pt=0  float_type=Single  exp_bits=8  fraction_bits=24  quantization=Truncate  overflow=Wrap  en=off  latency=1  pipeline=off  dbl_ovrd=off  block_type=convert
  io_delay : xbsIndex_r4/Delay  rst=off  infoeditControl=Selection of Reset will increase slice count due to use of real FFs and instead of SRLs  en=off  latency=0  reg_retiming=on  dbl_ovrd=off  block_type=delay
  reint1 : xbsIndex_r4/Reinterpret  force_arith_type=on  arith_type=Unsigned  force_bin_pt=on  bin_pt=0  block_type=reinterpret
  snap_tut_tge_gbe1_linkup_user_data_in : xbsIndex_r4/Gateway Out  inherit_from_input=off  hdl_port=on  rows=1  columns=1  UseAsDAC=off  DACChannel='1'  interface=None  automatic_assignment=on  address_offset=hex2dec('00')  intf_name=''  intf_description=''  timing_constraint=None  locs_specified=off  LOCs={}  io_standard={}  block_type=gatewayout
  sim_out : Outport
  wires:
  io_delay/1 -> cast_gw/1
  cast_gw/1 -> snap_tut_tge_gbe1_linkup_user_data_in/1
  snap_tut_tge_gbe1_linkup_user_data_in/1 -> sim_out/1
  out_reg/1 -> assert_reg/1
  assert_reg/1 -> reint1/1
  reint1/1 -> io_delay/1

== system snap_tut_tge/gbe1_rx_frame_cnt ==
  out_reg : Inport
  assert_reg : xbsIndex_r4/Assert  assert_type=on  type_source=Explicitly  gui_display_data_type=Fixed-point  arith_type=Unsigned  n_bits=32  bin_pt=0  preci_type=Single  exp_width=8  frac_width=24  assert_rate=off  rate_source=Explicitly  period=1  output_port=on  block_type=assert
  cast_gw : xbsIndex_r4/Convert  gui_display_data_type=Fixed-point  arith_type=Unsigned  n_bits=32  bin_pt=0  float_type=Single  exp_bits=8  fraction_bits=24  quantization=Truncate  overflow=Wrap  en=off  latency=1  pipeline=off  dbl_ovrd=off  block_type=convert
  io_delay : xbsIndex_r4/Delay  rst=off  infoeditControl=Selection of Reset will increase slice count due to use of real FFs and instead of SRLs  en=off  latency=0  reg_retiming=on  dbl_ovrd=off  block_type=delay
  reint1 : xbsIndex_r4/Reinterpret  force_arith_type=on  arith_type=Unsigned  force_bin_pt=on  bin_pt=0  block_type=reinterpret
  snap_tut_tge_gbe1_rx_frame_cnt_user_data_in : xbsIndex_r4/Gateway Out  inherit_from_input=off  hdl_port=on  rows=1  columns=1  UseAsDAC=off  DACChannel='1'  interface=None  automatic_assignment=on  address_offset=hex2dec('00')  intf_name=''  intf_description=''  timing_constraint=None  locs_specified=off  LOCs={}  io_standard={}  block_type=gatewayout
  sim_out : Outport
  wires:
  io_delay/1 -> cast_gw/1
  cast_gw/1 -> snap_tut_tge_gbe1_rx_frame_cnt_user_data_in/1
  snap_tut_tge_gbe1_rx_frame_cnt_user_data_in/1 -> sim_out/1
  out_reg/1 -> assert_reg/1
  assert_reg/1 -> reint1/1
  reint1/1 -> io_delay/1

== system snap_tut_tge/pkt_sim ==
  Constant : xbsIndex_r4/Constant  const=1  gui_display_data_type=Fixed-point  arith_type=Boolean  n_bits=16  bin_pt=14  preci_type=Single  exp_width=8  frac_width=24  explicit_period=on  period=1  equ=P=C  opselect=C  inp2=PCIN>>17  opr=+  inp1=P  carry=CIN  dbl_ovrd=off  block_type=constant
  Constant1 : xbsIndex_r4/Constant  const=0  gui_display_data_type=Fixed-point  arith_type=Boolean  n_bits=16  bin_pt=14  preci_type=Single  exp_width=8  frac_width=24  explicit_period=on  period=1  equ=P=C  opselect=C  inp2=PCIN>>17  opr=+  inp1=P  carry=CIN  dbl_ovrd=off  block_type=constant
  Constant2 : xbsIndex_r4/Constant  const=0  gui_display_data_type=Fixed-point  arith_type=Boolean  n_bits=16  bin_pt=14  preci_type=Single  exp_width=8  frac_width=24  explicit_period=on  period=1  equ=P=C  opselect=C  inp2=PCIN>>17  opr=+  inp1=P  carry=CIN  dbl_ovrd=off  block_type=constant
  Convert : xbsIndex_r4/Convert  gui_display_data_type=Fixed-point  arith_type=Boolean  n_bits=16  bin_pt=14  float_type=Single  exp_bits=8  fraction_bits=24  quantization=Truncate  overflow=Wrap  en=off  latency=0  pipeline=off  dbl_ovrd=off  block_type=convert
  Convert1 : xbsIndex_r4/Convert  gui_display_data_type=Fixed-point  arith_type=Boolean  n_bits=16  bin_pt=14  float_type=Single  exp_bits=8  fraction_bits=24  quantization=Truncate  overflow=Wrap  en=off  latency=0  pipeline=off  dbl_ovrd=off  block_type=convert
  Counter : xbsIndex_r4/Counter  cnt_type=Free Running  cnt_to=Inf  operation=Up  start_count=0  cnt_by_val=1  arith_type=Unsigned  n_bits=32  bin_pt=0  load_pin=off  rst=on  en=on  explicit_period=on  period=1  use_behavioral_HDL=off  implementation=Fabric  dbl_ovrd=off  block_type=counter
  Counter1 : xbsIndex_r4/Counter  cnt_type=Free Running  cnt_to=Inf  operation=Up  start_count=1  cnt_by_val=1  arith_type=Unsigned  n_bits=32  bin_pt=0  load_pin=off  rst=on  en=off  explicit_period=on  period=1  use_behavioral_HDL=off  implementation=Fabric  dbl_ovrd=off  block_type=counter
  Counter2 : xbsIndex_r4/Counter  cnt_type=Free Running  cnt_to=Inf  operation=Up  start_count=0  cnt_by_val=1  arith_type=Unsigned  n_bits=64  bin_pt=0  load_pin=off  rst=on  en=on  explicit_period=off  period=1  use_behavioral_HDL=off  implementation=Fabric  dbl_ovrd=off  block_type=counter
  Delay{,1..3} (4 alike) : xbsIndex_r4/Delay  rst=off  infoeditControl=Selection of Reset will increase slice count due to use of real FFs and instead of SRLs  en=off  latency=1  reg_retiming=on  dbl_ovrd=off  block_type=delay
  Inverter : xbsIndex_r4/Inverter  en=off  latency=0  dbl_ovrd=off  block_type=inv
  Mux : xbsIndex_r4/Mux  inputs=2  en=off  latency=1  precision=Full  arith_type=Unsigned  n_bits=16  bin_pt=14  quantization=Truncate  overflow=Wrap  dbl_ovrd=off  block_type=mux
  Mux1 : xbsIndex_r4/Mux  inputs=2  en=off  latency=1  precision=Full  arith_type=Unsigned  n_bits=16  bin_pt=14  quantization=Truncate  overflow=Wrap  dbl_ovrd=off  block_type=mux
  Mux2 : xbsIndex_r4/Mux  inputs=2  en=off  latency=1  precision=Full  arith_type=Unsigned  n_bits=16  bin_pt=14  quantization=Truncate  overflow=Wrap  dbl_ovrd=off  block_type=mux
  Relational : xbsIndex_r4/Relational  mode=a<b  op_type=Bool  en=off  latency=0  dbl_ovrd=off  block_type=relational
  Relational1 : xbsIndex_r4/Relational  mode=a>=b  op_type=Bool  en=off  latency=0  dbl_ovrd=off  block_type=relational
  eConst : Constant
  enable : Subsystem  Tag=xps:sw_reg  AncestorBlock=xps_library/Memory/software_register  mask(swreg){io_dir=From Processor, io_delay=0, init_val=0, sample_period=1, names=reg, bitwidths=32, bin_pts=0, arith_types=0, sim_port=on, show_format=off}
      mask prompts: io_dir "I/O direction"; io_delay "I/O delay"; init_val "Initial Value"; sample_period "Sample period"; names "Bitfield names [msb...lsb]"; bitwidths "Bitfield widths"; bin_pts "Bitfield binary pts"; arith_types "Bitfield types, ufix=0, fix=1, bool=2"; sim_port "Provide sim input/output?"; show_format "Print format string?"
      mask help: A 32-bit software-accessible register. Can be divided into bitfields of varying widths and types using the fields in the block mask.
      mask init:
      | swreg_init(gcb)
  enabler : xbsIndex_r4/Slice  nbits=1  boolean_output=off  mode=Lower Bit Location + Width  bit1=0  base1=MSB of Input  bit0=0  base0=LSB of Input  dbl_ovrd=off  block_type=slice
  negedge : Subsystem  AncestorBlock=casper_library_misc/edge_detect  mask(edge_detect){edge=Falling, polarity=Active High, x_in=[0 0.08 0.08 0.16 0.16 0.24 0.24 0.32 0.32 0.4], y_in=[-1 -1  1  1  1  1  1  1  1  1], x_out=[0.6 0.68 0.68 0.76 0.76 0.84 0.84 0.92 0.92 1], y_out=[-1 -1  1  1 -1 -1 -1 -1 -1 -1]}
      mask prompts: edge "Edge Type"; polarity "Output Polarity"; x_in "Input X Positions"; y_in "Input Y Positions"; x_out "Output X Positions"; y_out "Output Y Positions"
      mask help: Output is active for one-cycle after each edge of the specified type (i.e. rising, falling or both).
      mask init:
      | edge_detect_init(gcb,...
      |     'edge',edge,...
      |     'polarity',polarity,...
      |     'x_in',x_in,...
      |     'x_out',x_out,...
      |     'y_in',y_in,...
      |     'y_out',y_out);
      | 
      | x_in_num=str2num(getfield(getfield(get_param(gcb,'UserData'),'parameters'),'x_in'));
      | x_out_num=str2num(getfield(getfield(get_param(gcb,'UserData'),'parameters'),'x_out'));
      | y_in_num=str2num(getfield(getfield(get_param(gcb,'UserData'),'parameters'),'y_in'));
      | y_out_num=str2num(getfield(getfield(get_param(gcb,'UserData'),'parameters'),'y_out'));
  payload_len : Subsystem  Tag=xps:sw_reg  AncestorBlock=xps_library/Memory/software_register  mask(swreg){io_dir=From Processor, io_delay=0, init_val=0, sample_period=1, names=reg, bitwidths=32, bin_pts=0, arith_types=0, sim_port=on, show_format=off}
      mask prompts: io_dir "I/O direction"; io_delay "I/O delay"; init_val "Initial Value"; sample_period "Sample period"; names "Bitfield names [msb...lsb]"; bitwidths "Bitfield widths"; bin_pts "Bitfield binary pts"; arith_types "Bitfield types, ufix=0, fix=1, bool=2"; sim_port "Provide sim input/output?"; show_format "Print format string?"
      mask help: A 32-bit software-accessible register. Can be divided into bitfields of varying widths and types using the fields in the block mask.
      mask init:
      | swreg_init(gcb)
  period : Subsystem  Tag=xps:sw_reg  AncestorBlock=xps_library/Memory/software_register  mask(swreg){io_dir=From Processor, io_delay=0, init_val=0, sample_period=1, names=reg, bitwidths=32, bin_pts=0, arith_types=0, sim_port=on, show_format=off}
      mask prompts: io_dir "I/O direction"; io_delay "I/O delay"; init_val "Initial Value"; sample_period "Sample period"; names "Bitfield names [msb...lsb]"; bitwidths "Bitfield widths"; bin_pts "Bitfield binary pts"; arith_types "Bitfield types, ufix=0, fix=1, bool=2"; sim_port "Provide sim input/output?"; show_format "Print format string?"
      mask help: A 32-bit software-accessible register. Can be divided into bitfields of varying widths and types using the fields in the block mask.
      mask init:
      | swreg_init(gcb)
  posedge : Subsystem  AncestorBlock=casper_library_misc/edge_detect  mask(edge_detect){edge=Rising, polarity=Active High, x_in=[0 0.08 0.08 0.16 0.16 0.24 0.24 0.32 0.32 0.4], y_in=[-1 -1  1  1  1  1  1  1  1  1], x_out=[0.6 0.68 0.68 0.76 0.76 0.84 0.84 0.92 0.92 1], y_out=[-1 -1  1  1 -1 -1 -1 -1 -1 -1]}
      mask prompts: edge "Edge Type"; polarity "Output Polarity"; x_in "Input X Positions"; y_in "Input Y Positions"; x_out "Output X Positions"; y_out "Output Y Positions"
      mask help: Output is active for one-cycle after each edge of the specified type (i.e. rising, falling or both).
      mask init:
      | edge_detect_init(gcb,...
      |     'edge',edge,...
      |     'polarity',polarity,...
      |     'x_in',x_in,...
      |     'x_out',x_out,...
      |     'y_in',y_in,...
      |     'y_out',y_out);
      | 
      | x_in_num=str2num(getfield(getfield(get_param(gcb,'UserData'),'parameters'),'x_in'));
      | x_out_num=str2num(getfield(getfield(get_param(gcb,'UserData'),'parameters'),'x_out'));
      | y_in_num=str2num(getfield(getfield(get_param(gcb,'UserData'),'parameters'),'y_in'));
      | y_out_num=str2num(getfield(getfield(get_param(gcb,'UserData'),'parameters'),'y_out'));
  sim_freq : Constant  Value=200
  sim_length : Constant  Value=50
  d_out : Outport
  valid : Outport  Port=2
  eof : Outport  Port=3
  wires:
  Counter/1 -> Relational/1
  sim_length/1 -> payload_len/1(sim_1)
  posedge/1(out) -> Counter/1
  Mux2/1 -> eof/1
  Mux1/1 -> valid/1
  Delay3/1 -> d_out/1
  Counter2/1 -> Delay3/1
  enabler/1 -> Mux1/1, Mux2/1, Convert1/1
  enable/1(in_reg) -> enabler/1
  eConst/1 -> enable/1(sim_1)
  Convert1/1 -> Inverter/1
  Inverter/1 -> Counter2/1
  Delay2/1 -> Counter2/2
  Convert/1 -> Mux2/3
  Constant2/1 -> Mux1/2, Mux2/2
  Mux/1 -> Mux1/3
  Delay1/1 -> Mux/1
  Constant/1 -> Mux/3
  Constant1/1 -> Mux/2
  Delay/1 -> Convert/1
  negedge/1(out) -> Delay/1
  Relational1/1 -> posedge/1(in), Counter1/1
  Counter1/1 -> Relational1/1
  period/1(in_reg) -> Relational1/2
  sim_freq/1 -> period/1(sim_1)
  Relational/1 -> negedge/1(in), Counter/2, Delay1/1, Delay2/1
  payload_len/1(in_reg) -> Relational/2
